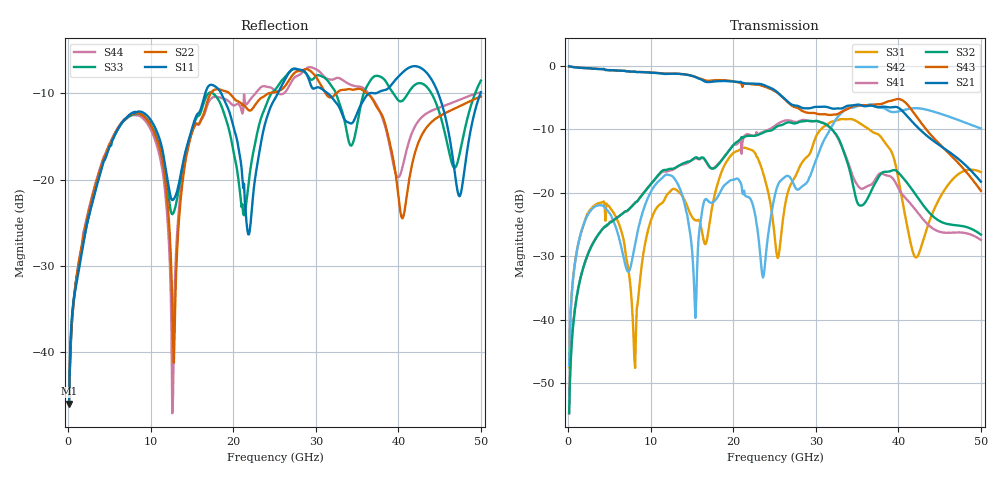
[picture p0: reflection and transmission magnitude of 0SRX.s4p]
! DAC39RF10ACK
! 256-pin FCBGA package
! Texas Instruments 8/20/2022
! Single-ended  S-parameters
! PORT#  PORT_NAME  NET_NAME
! PORT1:  xSRXN.DIEBUMP  xSRXN
! PORT2:  xSRXN.BGA  xSRXN
! PORT3:  xSRXP.DIEBUMP  xSRXP
! PORT4:  xSRXP.BGA  xSRXP
! Touchstone Ver. 1.0
! Number of ports is 4
# Hz	S	MA	R	50.000000
! SCATTERING PARAMETERS  :
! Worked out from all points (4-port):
!   500 points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, 100 MHz to 50 GHz, reference 50 ohm
!   strongest paths, dB at 100 MHz, 12.6 GHz, 25.1 GHz, 37.6 GHz, 50 GHz:
!     S21: 0.0, -1.2, -3.9, -6.5, -18.3
!     S43: -0.1, -1.2, -4.0, -6.0, -19.7
!     S32: -54.7, -16.2, -9.7, -17.5, -26.6
!     S41: -54.8, -16.4, -9.4, -17.1, -27.4
!     S42: -47.3, -17.4, -20.0, -6.5, -9.9
!     S31: -47.5, -19.5, -28.0, -10.8, -16.7
!   lowest |S11| = -46.0 dB at 100 MHz (marker M1), VSWR 1.01, Z = 50.4 + j0.338 ohm
!   |S11| at or under -10 dB: start of sweep to 16.6 GHz; 18.53 GHz to 25.39 GHz (6.852 GHz wide, 31.2 % of centre); 44.83 GHz to 49.95 GHz (5.116 GHz wide, 10.8 % of centre)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
1e8  0.005036 41.8  0.9893 -2.6  0.003139 64.8  0.002051 -107.9
     0.9956 -2.5  0.005226 34.3  0.001968 -98.4  0.004236 83.5
     0.004214 83.2  0.00183 -111.4  0.006412 19.9  0.9918 -2.8
     0.001827 -99.2  0.004309 83.3  0.9889 -2.5  0.005446 38.6
3.6e9  0.09754 25.0  0.9463 -80.0  0.08258 6.5  0.04631 178.2
       0.9455 -80.0  0.1045 -23.2  0.04699 178.3  0.07973 6.5
       0.08251 6.4  0.04645 178.3  0.1013 26.4  0.9452 -80.5
       0.0464 178.1  0.07954 6.6  0.9497 -80.5  0.1068 -23.9
8e9  0.2429 -61.8  0.8818 -175.6  0.005122 -3.3  0.081 91.9
     0.9015 -175.4  0.2423 -110.8  0.08264 91.8  0.0364 149.9
     0.004943 -29.7  0.0816 91.5  0.2396 -62.1  0.8999 -176.6
     0.08244 92.2  0.03651 151.7  0.9011 -176.5  0.2367 -112.5
1.26e10  0.07608 -98.0  0.8667 85.1  0.1082 -24.6  0.152 -13.4
         0.867 85.0  0.01905 126.3  0.1545 -14.6  0.1353 20.4
         0.1065 -25.0  0.1543 -15.0  0.06302 -94.8  0.8692 83.0
         0.1509 -12.9  0.1351 20.6  0.8694 82.9  0.004421 174.4
1.57e10  0.2418 -76.0  0.7984 13.8  0.05983 -178.3  0.1878 -89.0
         0.8002 13.8  0.2101 -80.1  0.1885 -90.3  0.03467 88.0
         0.06099 -177.7  0.1875 -91.0  0.2334 -76.6  0.8063 11.9
         0.1856 -88.5  0.03506 86.3  0.8056 11.9  0.2086 -84.3
2.38e10  0.2072 -34.3  0.7034 -163.6  0.1315 -99.3  0.3043 94.2
         0.7031 -163.9  0.3058 -126.5  0.3016 90.5  0.02444 162.9
         0.1296 -98.3  0.3016 90.7  0.2578 -37.2  0.6844 -168.7
         0.3057 93.9  0.02587 162.0  0.6867 -168.5  0.348 -130.1
5e10  0.3212 -75.6  0.13 26.0  0.1183 -93.8  0.03633 -93.3
      0.1223 36.3  0.3038 -128.1  0.03713 -100.0  0.3043 -30.1
      0.1459 -91.8  0.04683 -116.3  0.3754 -79.9  0.1195 10.4
      0.04253 -110.8  0.3214 -28.7  0.1037 15.4  0.3214 -132.6
